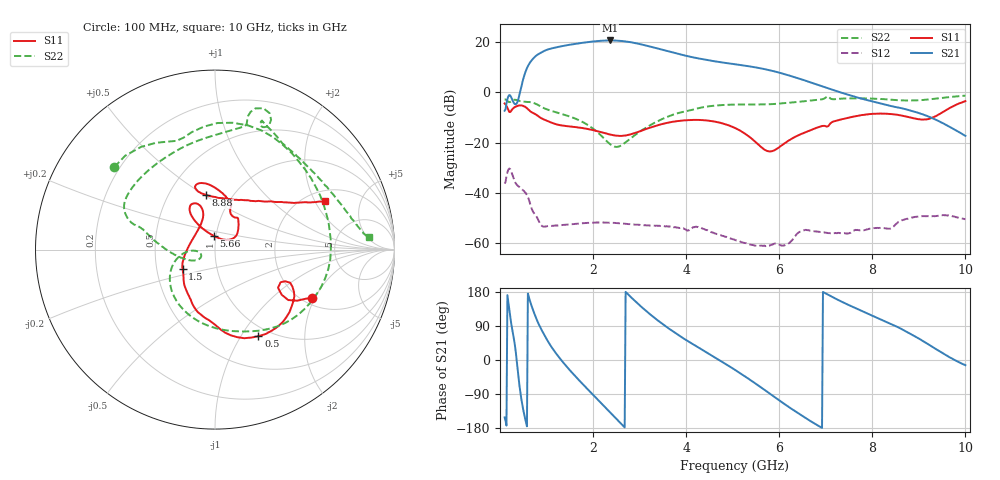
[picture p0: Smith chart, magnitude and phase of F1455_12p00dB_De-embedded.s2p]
! Integrated Device Technology
! Corporate Headquarters
! 6024 Silver Creek Valley Road
! San Jose, CA 95138  USA
! Phone:  1-408-284-8200
! Toll Free:  1-800-223-1366
! Webpage:  http://www.idt.com/
! Timing and RF Division
! 515 Groton Road, Suite 102
! Westford, MA 01886-6024
! Device:  F1455
! Description: 6-bit 0.5 dB Transmit Variable Gain Amplifier
! Frequency:  1400.0 -  2300.00 MHz
! Package:  6x6 mm Thin QFN Plastic Package: 28 pin
! State:  24
! Atten State:  12.0 dB
! Voltage:  +5.00 Volts
! Current:  217.666 mA
! Data:  The device was measured on a the F1455 evaluation board which has
!  individual transmission lines to the RF pins.  Data was collected
!  using a calibrated network analyzer.  The evaluation board was
!  de-embedded using a TRL calibration technique.
!  The reference plane is the edge of the package pin.
!  Pin  1 = CSb
!  Pin  2 = DATA
!  Pin  3 = CLK
!  Pin  4 = RSET
!  Pin  5 = GND
!  Pin  6 = RFIN  = Port 1
!  Pin  7 = GND
!  Pin  8 = NC
!  Pin  9 = NC
!  Pin 10 = NC
!  Pin 11 = NC
!  Pin 12 = NC
!  Pin 13 = NC
!  Pin 14 = /STBY
!  Pin 15 = GND
!  Pin 16 = RFOUT  = Port 2
!  Pin 17 = GND
!  Pin 18 = NC
!  Pin 19 = NC
!  Pin 20 = NC
!  Pin 21 = GND
!  Pin 22 = NC
!  Pin 23 = GND
!  Pin 24 = NC
!  Pin 25 = NC
!  Pin 26 = NC
!  Pin 27 = GND
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# GHz S dB R 50
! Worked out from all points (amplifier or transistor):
!   496 points, 100 MHz to 10 GHz, reference 50 ohm
!   highest |S21| = 20.7 dB at 2.36 GHz (marker M1)
!   |S21| within 3 dB of that: 1.147 GHz to 3.347 GHz (2.2 GHz wide, 97.9 % of centre)
!   unconditionally stable (mu >= 1): start of sweep to end of sweep
!   at 1.74 GHz: K = 18.50, MAG = 20.2 dB, |S12| = -52.0 dB
!   at 5.06 GHz: K = 76.50, MAG = 13.1 dB, |S12| = -58.7 dB
!   at 10 GHz: K = 170.34, MAG = -8.7 dB, |S12| = -50.4 dB
!   S11 on the Smith chart (normalised r, x): 100 MHz: 2.24, -1.90; 500 MHz: 0.88, -1.19; 1.5 GHz: 0.68, -0.15; 5.66 GHz: 0.98, +0.15; 8.88 GHz: 0.76, +0.51; 10 GHz: 2.46, +2.44
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0.1  -4.38 -26.5  -7.28 -151.4  -36.21 45.6  -2.79 140.7
0.38  -5.32 -40.1  -3.58 -24.0  -37.03 -113.6  -3.16 57.0
0.5  -5.36 -63.4  5.37 -131.1  -38.94 -151.4  -3.62 27.4
0.68  -7.85 -92.6  12.75 142.5  -46.13 146.4  -3.95 -14.6
0.8  -9.11 -107.8  14.93 103.7  -49.82 130.1  -4.78 -42.4
0.94  -10.71 -121.0  16.41 69.0  -53.37 124.4  -6.21 -68.6
1.22  -12.72 -139.4  17.99 15.0  -52.94 95.9  -7.96 -107.5
1.5  -13.52 -149.2  18.98 -26.8  -52.48 68.5  -9.56 -136.5
1.76  -14.10 -157.0  19.72 -61.3  -51.99 48.4  -11.58 -156.8
2.06  -15.21 -168.5  20.39 -99.4  -51.74 28.7  -15.26 -173.8
2.36  -16.69 171.3  20.68 -137.6  -51.82 11.0  -20.46 -173.1
2.56  -17.25 152.3  20.55 -162.9  -52.03 0.7  -21.46 -154.9
2.76  -16.90 132.9  20.13 172.4  -52.35 -8.0  -18.97 -149.7
3.06  -15.08 113.7  19.02 138.0  -52.76 -19.1  -14.92 -163.3
3.4  -12.98 107.6  17.43 103.7  -53.04 -30.9  -11.35 179.9
4.1  -10.96 114.8  14.15 45.1  -54.17 -49.3  -7.04 163.3
5.06  -14.22 124.9  11.20 -26.8  -58.71 -90.9  -4.82 148.1
5.66  -22.44 93.7  9.38 -76.8  -61.01 -89.2  -4.75 124.0
6.7  -14.83 44.1  3.85 -163.3  -54.98 -135.5  -3.17 78.3
8.36  -8.52 106.6  -5.24 97.1  -54.20 159.9  -2.82 62.3
8.88  -10.25 99.3  -7.49 64.9  -49.68 143.1  -3.18 41.8
10  -3.46 23.9  -17.25 -13.7  -50.43 68.5  -1.29 4.6
